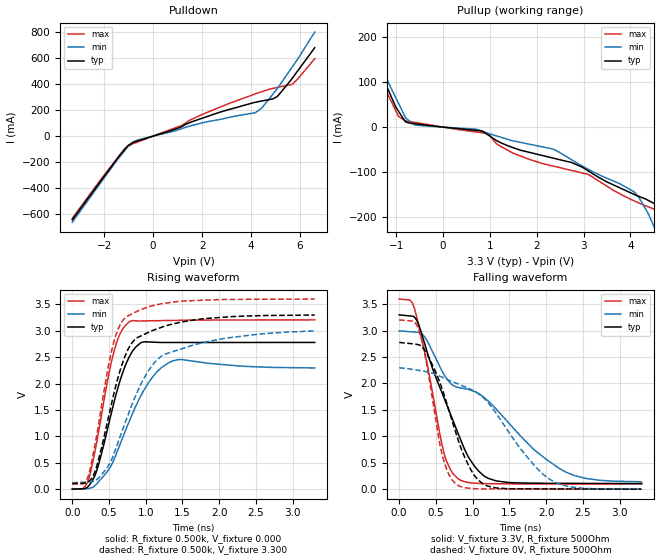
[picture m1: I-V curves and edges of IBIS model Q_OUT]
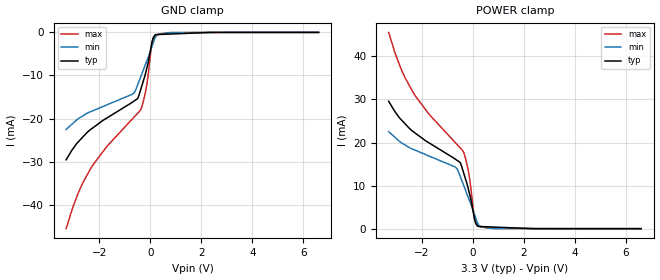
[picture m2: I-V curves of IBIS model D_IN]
|Texas Instruments Incorporated
|3.3V Differential PECL/LVDS to TTL translator
| Marketing part#   Voltage Range   Package-type   #pins
|SN65EPT21DGK   3.0 to 3.6 V   MSOP   8
|SN65EPT21DGKR   3.0 to 3.6 V   MSOP   8
|SN65EPT21D   3.0 to 3.6 V   SOIC   8
|SN65EPT21DR   3.0 to 3.6 V   SOIC   8
[IBIS Ver]   4.0
[File name]   sn65ept21.ibs
[File Rev]   1.0
[Date]   02/17/2011
[Source]   Texas Instruments Incorporated.
   Analog-eLab, HPA
   12500 TI Blvd
   Dallas, TX -75243
   For Support e-mail: elab_ibis@list.ti.com
[Notes]   Revision History:
   1.0: 02/17/2011
   - Initial version of the model
   - Initial Model generated from simulations.
   - Model not matched to measurements
[Disclaimer]
 This product is designed as an aid for customers of Texas Instruments.
 No warranties, either expressed or implied, with respect to this third
 party software (if any) or with respect to its fitness for any
 particular purpose is claimed by Texas Instruments or the author. The
 software (if any) is provided solely on an "as is" basis. The entire
 risk as to its quality and performance is with the customer
[Copyright] (C) Copyright 2011 Texas Instruments Incorporated.
   All rights reserved.
|   TSC2003
[Component]   sn65ept21
[Manufacturer] TI
[Package]   | 8 MSOP  package
| variable   typ   min   max
R_pkg   0.094875   0.04725   0.12179
L_pkg   1.66309nH   1.49206nH   1.83822nH
C_pkg   0.407492pF   0.39032pF   0.42729pF
|-------------------------PIN------------------------------------------------
[Pin] signal_name  model_name   R_pin   L_pin   C_pin
1   NC   NC   0.01106   0.75153nH   0.31231pF
2   D   D_IN   0.11188   1.70889nH   0.40172pF
3   D-   D_IN   0.11188   1.70869nH   0.40652pF
4   VBB   TERM   0.12179   1.83822nH   0.39032pF
5   GND   GND   0.04725   1.49206nH   0.42729pF
6   NC   NC   0.01106   0.73982nH   0.33464pF
7   Q   Q_OUT   0.11187   1.70867nH   0.40482pF
8   VCC   POWER   0.06458   1.52205nH   0.41428pF
[Diff_pin]   inv_pin   vdiff   tdelay_typ   tdelay_min   tdelay_max
2   3   200mV   NA   NA   NA
|   TERM Model
[Model] TERM
Model_type Terminator
C_comp   0   0   0
| variable   typ   min   max
[Voltage Range]   3.3V   3.0V   3.6V
[POWER Clamp Reference]  3.3V   3.0V   3.6V
[GND Clamp Reference]   0.0V   0.0V   0.0V
|Operating Temperature
[Temperature Range]   27   125   -40
| Models and submodels in the file (3): Q_OUT (Output), D_IN (Input), TERM (Terminator)
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|   Q_OUT
[Model]   Q_OUT
Model_type   Output
Polarity   Non-Inverting
Vmeas = 1.65
Vref = 1.65
Cref = 20pF
Rref = 500
|   typ   min   max
C_comp   1.41416pF   1.25330pF   1.50236pF
[Voltage Range]   3.3   3   3.6
[Temperature Range]   27   125   -40
[Pullup Reference]   3.3   3   3.6
[Pulldown Reference]   -0   -0   -0
[Power Clamp Reference]   3.3   3   3.6
[GND Clamp Reference]   -0   -0   -0
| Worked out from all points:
|   slope of the pulldown table from 0 to 0.495 V, typ, clamps not added: 17 ohm
|   slope of the pullup table from 0 to 0.495 V, typ, clamps not added: 97.5 ohm
|   falling waveform, V_fixture 3.3V, R_fixture 500Ohm: 20-80 % time 526ps typ, 1.35ns min, 293ps max; typ from 3.3 V to 0.107 V
|   rising waveform, R_fixture 0.500k, V_fixture 0.000: 20-80 % time 316ps typ, 426ps min, 261ps max; typ from 0.002 V to 2.78 V
|   rising waveform, R_fixture 0.500k, V_fixture 3.300: 20-80 % time 372ps typ, 561ps min, 285ps max; typ from 0.109 V to 3.3 V
|   falling waveform, V_fixture 0V, R_fixture 500Ohm: 20-80 % time 414ps typ, 789ps min, 239ps max; typ from 2.77 V to 0 V
[Pulldown]
|   Voltage   I(typ)   I(min)   I(max)
-3.3V     -643.7mA   -662.9mA   -633.3mA
-1.135V   -97.89mA   -106.3mA   -90.89mA
-803.2mV  -48.02mA   -42.31mA   -57.34mA
-617.3mV  -36.91mA   -28.83mA   -44.1mA
1.19V     75.44mA    59.04mA    84.25mA
1.992V    137mA      101.5mA    165.1mA
4.176V    260.8mA    180.8mA    326.5mA
4.428V    270.3mA    214.3mA    341.8mA
4.898V    286.8mA    325.2mA    368.1mA
5.068V    305.8mA    366.4mA    374.8mA
5.695V    448.9mA    536.3mA    401.4mA
6.6V      681.2mA    801.3mA    596.4mA
[Pullup]
|   Voltage   I(typ)   I(min)   I(max)
-3.3V     641.1mA    700mA      615.4mA
-1.754V   230.1mA    249.3mA    219.2mA
-951.8mV  34.95mA    52.37mA    23.54mA
-782.3mV  10.77mA    18.99mA    13.72mA
933.6mV   -15.49mA   -12.82mA   -14.27mA
1.453V    -44.07mA   -29.44mA   -55.72mA
2.389V    -69.82mA   -50.6mA    -87.48mA
4.076V    -149.3mA   -143.5mA   -163.6mA
4.589V    -173.9mA   -240mA     -185.8mA
4.96V     -243.5mA   -329mA     -201.2mA
5.18V     -295.9mA   -386.5mA   -223.2mA
6.6V      -654.1mA   -756.6mA   -562.3mA
[Ramp]
R_load = 500
|   typ   min   max
dV/dt_r   1.6659/3.15449e-010   1.37668/4.26283e-010   1.92179/2.60773e-010
dV/dt_f   1.91409/5.27048e-010   1.71305/1.3506e-009   2.09884/2.92035e-010
[Falling Waveform]
V_fixture = 3.3V
V_fixture_min = 3V
V_fixture_max = 3.6V
R_fixture = 500Ohm
C_fixture = 0F
|   Time   V(typ)   V(min)   V(max)
0s        3.297V     2.994V     3.596V
204.4ps   3.257V     2.972V     3.432V
344.3ps   2.765V     2.884V     2.61V
607.6ps   1.736V     2.173V     698mV
797.9ps   1.07V      1.926V     201mV
1.023ns   441.2mV    1.849V     113.6mV
1.32ns    156.2mV    1.514V     102.8mV
1.817ns   114.5mV    771mV      98.33mV
2.268ns   109.6mV    323mV      98.07mV
3.3ns     106.5mV    139.3mV    97.48mV
[Rising Waveform]
R_fixture = 0.500k
V_fixture = 0.000
V_fixture_min = 0.000
V_fixture_max = 0.000
C_fixture = 0.000
|  time   V(typ)   V(min)   V(max)
0s        2.261mV    1.365mV    2.844mV
180.5ps   18.04mV    12.36mV    65.16mV
300ps     234mV      59.26mV    652.6mV
567.4ps   1.641V     561.9mV    2.608V
657.3ps   2.086V     875.4mV    2.961V
771.3ps   2.495V     1.271V     3.166V
928ps     2.768V     1.755V     3.185V
1.093ns   2.785V     2.124V     3.189V
1.378ns   2.778V     2.434V     3.196V
3.3ns     2.779V     2.296V     3.206V
[Rising Waveform]
R_fixture = 0.500k
V_fixture = 3.300
V_fixture_min = 3.000
V_fixture_max = 3.600
C_fixture = 0.000
|  time   V(typ)   V(min)   V(max)
0s        108.7mV    124.8mV    100.3mV
192.4ps   120.4mV    134.4mV    166.7mV
300ps     303.4mV    150.5mV    769.5mV
545.6ps   1.69V      596.2mV    2.684V
635.6ps   2.176V     936.4mV    3.069V
727.5ps   2.549V     1.291V     3.258V
981.3ps   2.933V     2.114V     3.423V
1.257ns   3.087V     2.554V     3.521V
2.121ns   3.262V     2.866V     3.593V
3.3ns     3.298V     2.998V     3.6V
[Falling Waveform]
|Gnd
V_fixture = 0V
V_fixture_min = 0V
V_fixture_max = 0V
R_fixture = 500Ohm
C_fixture = 0F
|   Time   V(typ)   V(min)   V(max)
0s        2.775V     2.295V     3.201V
264.1ps   2.732V     2.247V     3.02V
372.5ps   2.576V     2.22V      2.384V
578.2ps   1.925V     2.121V     689.3mV
675.4ps   1.501V     2.062V     281.1mV
779.5ps   1.034V     2.002V     90.46mV
957.4ps   411.7mV    1.899V     17.3mV
1.146ns   97.04mV    1.73V      5.664mV
2.06ns    4.985mV    177.7mV    3.26mV
3.3ns     29.37uV    2.662mV    -873.2nV
|   D_IN
[Model]   D_IN
Model_type   Input
Vinl = 1.515
Vinh = 2.247
|   typ   min   max
C_comp   0.38080pF   0.32668pF   0.43327pF
[Voltage Range]   3.3   3   3.6
[Temperature Range]   27   125   -40
[Power Clamp Reference]   3.3   3   3.6
[GND Clamp Reference]   -0   -0   -0
[GND Clamp]
|   Voltage   I(typ)   I(min)   I(max)
-3.3V     -29.59mA   -22.52mA   -45.58mA
-2.842V   -25.53mA   -20.1mA    -37.53mA
-2.333V   -22.52mA   -18.4mA    -31.58mA
-1.698V   -19.85mA   -16.82mA   -26.45mA
-699.7mV  -16.19mA   -14.35mA   -20.07mA
-500.6mV  -15.39mA   -12.25mA   -18.81mA
-349.3mV  -12.75mA   -9.909mA   -17.62mA
-135.1mV  -8.246mA   -6.587mA   -12.04mA
68.48mV   -2.247mA   -3.236mA   -2.381mA
195.6mV   -565uA     -1.207mA   -717.9uA
794mV     -376.7uA   -38.61uA   -75.35uA
6.6V      0A         0A         0A
[POWER Clamp]
|   Voltage   I(typ)   I(min)   I(max)
-3.3V     29.59mA    22.52mA    45.58mA
-2.842V   25.53mA    20.1mA     37.53mA
-2.333V   22.52mA    18.4mA     31.58mA
-1.698V   19.85mA    16.82mA    26.45mA
-699.7mV  16.19mA    14.35mA    20.07mA
-500.6mV  15.39mA    12.25mA    18.81mA
-349.3mV  12.75mA    9.909mA    17.62mA
-135.1mV  8.246mA    6.587mA    12.04mA
68.48mV   2.247mA    3.236mA    2.381mA
195.6mV   565uA      1.207mA    717.9uA
794mV     376.7uA    38.61uA    75.35uA
6.6V      0A         0A         0A
